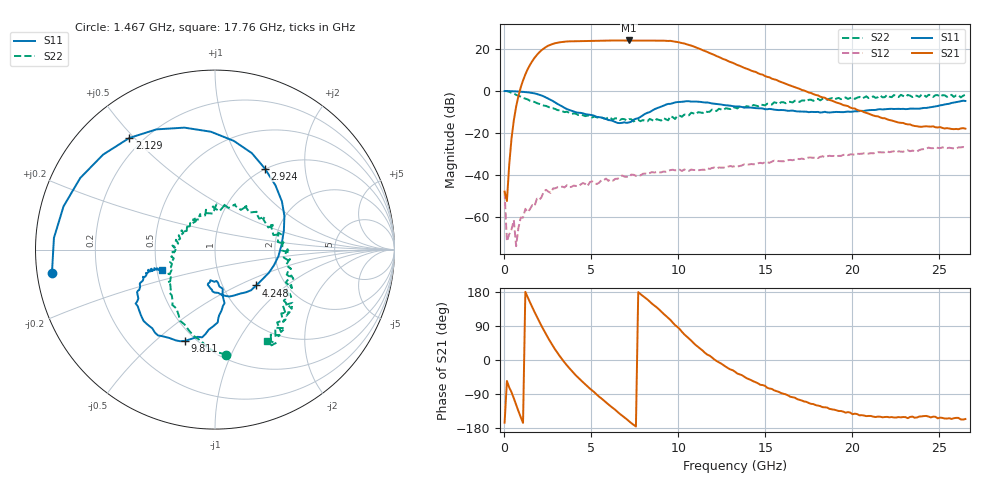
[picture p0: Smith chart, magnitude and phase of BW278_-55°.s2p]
!Agilent Technologies,N5242A,MY52422126,A.09.90.01
!Agilent N5242A: A.09.90.01
!Date: Thursday, January 16, 2014 00:29:51
!Correction: S11(Full 2 Port with power(1,2))
!S21(Full 2 Port with power(1,2))
!S12(Full 2 Port with power(1,2))
!S22(Full 2 Port with power(1,2))
!S2P File: Measurements: S11, S21, S12, S22:
# Hz S  dB  R 50
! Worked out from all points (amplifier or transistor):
!   201 points, 10 MHz to 26.5 GHz, reference 50 ohm
!   highest |S21| = 24.1 dB at 7.162 GHz (marker M1)
!   |S21| within 3 dB of that: 2.413 GHz to 10.92 GHz (8.503 GHz wide, 128 % of centre)
!   unconditionally stable (mu >= 1): 153 MHz to end of sweep
!   at 4.381 GHz: K = 4.70, MAG = 24.5 dB, |S12| = -44.6 dB
!   at 13.26 GHz: K = 4.88, MAG = 14.5 dB, |S12| = -35.8 dB
!   at 26.5 GHz: K = 18.06, MAG = -11.1 dB, |S12| = -27.0 dB
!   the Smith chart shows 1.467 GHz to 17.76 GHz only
!   S11 on the Smith chart (normalised r, x): 1.467 GHz: 0.04, -0.07; 2.129 GHz: 0.15, +0.48; 2.924 GHz: 0.99, +1.25; 4.248 GHz: 1.43, -0.63; 9.811 GHz: 0.44, -0.63; 17.76 GHz: 0.53, -0.13
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1e7  -0.02 -1.4  -47.89 -165.3  -47.97 80.5  -0.00 -0.8
1.0696e9  -0.40 -133.6  5.06 -166.0  -60.34 -125.0  -3.28 -67.6
1.46695e9  -0.75 -171.8  12.43 152.3  -56.33 -166.6  -4.62 -84.0
1.8643e9  -1.41 152.0  17.19 114.5  -51.28 145.2  -5.76 -98.6
2.1292e9  -2.11 127.5  19.43 90.2  -50.64 122.7  -6.43 -107.2
2.52655e9  -3.65 92.0  21.65 56.9  -47.95 108.6  -7.55 -118.7
2.9239e9  -5.51 58.3  22.82 27.2  -46.34 101.0  -8.56 -129.1
3.58615e9  -8.58 4.4  23.63 -13.8  -44.92 82.6  -9.86 -145.5
4.2484e9  -10.33 -40.9  23.76 -47.0  -45.20 66.6  -11.44 -154.7
4.5133e9  -10.63 -53.9  23.81 -58.5  -43.81 75.1  -11.53 -158.1
5.70535e9  -12.99 -94.4  24.01 -106.4  -42.56 62.3  -13.00 -177.3
7.1623e9  -14.97 -86.2  24.11 -161.5  -41.00 50.0  -13.37 149.9
8.08945e9  -10.84 -80.2  24.05 164.3  -39.29 33.9  -14.15 134.1
8.88415e9  -7.83 -87.9  23.99 133.7  -38.80 28.7  -13.74 115.2
9.8113e9  -5.43 -108.2  23.52 92.0  -37.78 21.4  -13.34 83.5
1.03411e10  -4.97 -121.1  22.65 67.7  -37.35 14.9  -11.18 65.9
1.100335e10  -5.00 -135.0  20.80 39.2  -37.65 6.1  -10.99 47.1
1.206295e10  -6.03 -149.8  17.22 1.6  -36.44 2.2  -9.38 23.6
1.3255e10  -7.34 -158.1  12.93 -30.9  -35.80 -5.6  -7.87 0.3
1.77583e10  -9.99 -159.1  -1.44 -116.3  -31.83 -41.6  -4.68 -60.5
2.212915e10  -8.50 -146.9  -13.81 -151.3  -29.15 -85.8  -2.68 -91.6
2.65e10  -4.72 -148.4  -17.94 -155.7  -26.97 -137.1  -1.66 -121.3
